ORGANIZATION_BLOCK OB 100
BEGIN
	L		MD 0
	__ASSERT==	__ACCU 1,	0
	L		100
	T		MD 0
END_ORGANIZATION_BLOCK



ORGANIZATION_BLOCK OB 1
BEGIN
	// assert 4-accus
	__FEATURE	0
	__ASSERT==	__ACCU 1,	4

	// check that OB 100 was executed
	L		MD 0
	__ASSERT==	__ACCU 1,	100


	CALL SFC 46 // STOP CPU
END_ORGANIZATION_BLOCK
